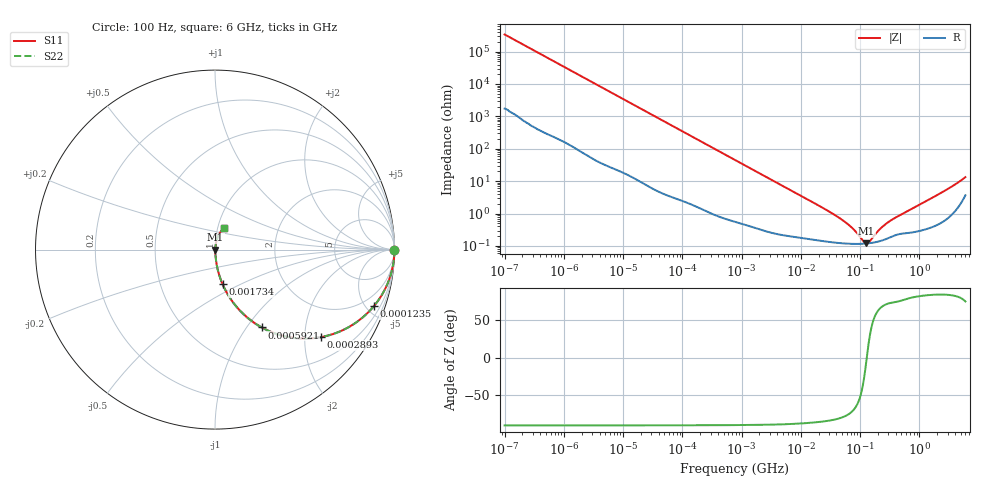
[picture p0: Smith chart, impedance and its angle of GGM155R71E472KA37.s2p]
!Murata Part Number: GGM155R71E472KA37
!These Parameters are Measured in Series Mode Connection
!Data Generated on Jun 19, 2026
!  o--ll--o
!Port1  Port2
!  o------o
!Operation Temp=25[degC], DC Bias Voltage=0[V]
!Freq. Start=100[Hz] Stop=6[GHz] 401[Steps]
# Hz S RI R 50
!Freq.(Hz) S11(Real) S11(Imag) S21(Real) S21(Imag) S12(Real) S12(Imag) S22(Real) S22(Imag)
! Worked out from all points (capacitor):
!   401 points, 100 Hz to 6 GHz, reference 50 ohm
!   read as one part in series: C = 4.68 nF near 109 Hz
!   lowest |Z| = 119 mohm at 127.6 MHz (marker M1)
!   series resonance near 129.9 MHz, so ESL is about 320 pH
!   S11 on the Smith chart (normalised r, x): 100 Hz: open; 123.5 kHz: 1.04, -5.61; 289.3 kHz: 1.02, -2.41; 592.1 kHz: 1.01, -1.18; 1.734 MHz: 1.01, -0.41; 6 GHz: 1.07, +0.26
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100  1 -0.000295  1.6e-06 0.000295  1.6e-06 0.000295  1 -0.000295
2008  0.9999 -0.00587  6.13e-05 0.00587  6.13e-05 0.00587  0.9999 -0.00587
12592  0.9985 -0.0365  0.00154 0.0365  0.00154 0.0365  0.9985 -0.0365
40335  0.9859 -0.1151  0.0141 0.1151  0.0141 0.1151  0.9859 -0.1151
123542  0.8855 -0.3146  0.1145 0.3146  0.1145 0.3146  0.8855 -0.3146
184852  0.7776 -0.4118  0.2224 0.4118  0.2224 0.4118  0.7776 -0.4118
289253  0.591 -0.4873  0.409 0.4873  0.409 0.4873  0.591 -0.4873
413847  0.4161 -0.4882  0.5839 0.4882  0.5839 0.4882  0.4161 -0.4882
592111  0.2605 -0.4335  0.7395 0.4335  0.7395 0.4335  0.2605 -0.4335
774597  0.1724 -0.3716  0.8276 0.3716  0.8276 0.3716  0.1724 -0.3716
1734173  0.0427 -0.1936  0.9573 0.1936  0.9573 0.1936  0.0427 -0.1936
4440638  0.0085 -0.0788  0.9915 0.0788  0.9915 0.0788  0.0085 -0.0788
1.555665e7  0.0021 -0.0227  0.9979 0.0227  0.9979 0.0227  0.0021 -0.0227
5.699437e7  0.00121 -0.0052  0.9988 0.0052  0.9988 0.0052  0.00121 -0.0052
8.154455e7  0.00116 -0.00274  0.9988 0.00274  0.9988 0.00274  0.00116 -0.00274
1.166697e8  0.00117 -0.000611  0.9988 0.000611  0.9988 0.000611  0.00117 -0.000611
1.275994e8  0.00119 -0.000101  0.9988 0.000101  0.9988 0.000101  0.00119 -0.000101
1.459435e8  0.00122 0.000662  0.9988 -0.000662  0.9988 -0.000662  0.00122 0.000662
2.183701e8  0.00142 0.00305  0.9986 -0.00305  0.9986 -0.00305  0.00142 0.00305
3.124326e8  0.00182 0.00543  0.9982 -0.00543  0.9982 -0.00543  0.00182 0.00543
1.95892e9  0.00562 0.0358  0.9944 -0.0358  0.9944 -0.0358  0.00562 0.0358
6e9  0.0499 0.1178  0.9501 -0.1178  0.9501 -0.1178  0.0499 0.1178
